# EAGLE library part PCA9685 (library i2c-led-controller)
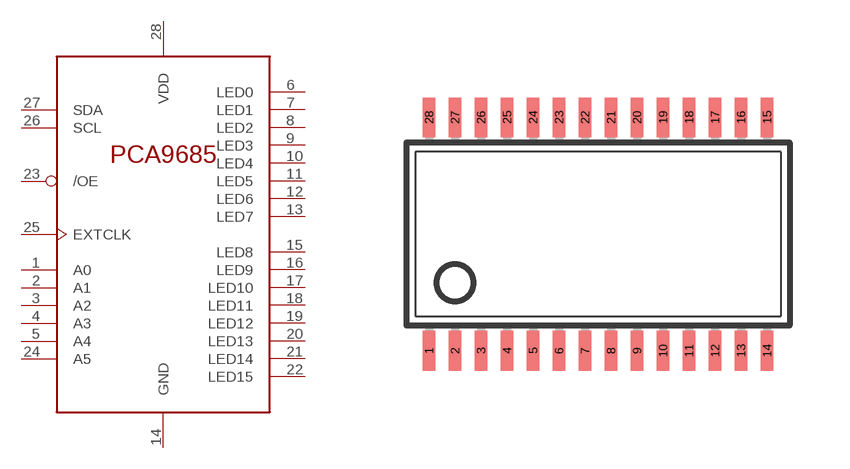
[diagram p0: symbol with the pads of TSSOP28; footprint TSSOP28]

Designator prefix -

## PCA9685PW  [TSSOP28]
1  A0
2  A1
3  A2
4  A3
5  A4
6  LED0
7  LED1
8  LED2
9  LED3
10  LED4
11  LED5
12  LED6
13  LED7
14  GND  pwr
15  LED8
16  LED9
17  LED10
18  LED11
19  LED12
20  LED13
21  LED14
22  LED15
23  /OE
24  A5
25  EXTCLK  in
26  SCL
27  SDA
28  VDD  pwr

## Footprint TSSOP28 (pad centres in mm)
smd 0.305 x 0.991: 1 -4.225,-2.918; 2 -3.575,-2.918; 3 -2.925,-2.918; 4 -2.275,-2.918; 5 -1.625,-2.918; 6 -0.975,-2.918; 7 -0.325,-2.918; 8 0.325,-2.918; 9 0.975,-2.918; 10 1.625,-2.918; 11 2.275,-2.918; 12 2.925,-2.918; 13 3.575,-2.918; 14 4.225,-2.918; 15 4.225,2.918; 16 3.575,2.918; 17 2.925,2.918; 18 2.275,2.918; 19 1.625,2.918; 20 0.975,2.918; 21 0.325,2.918; 22 -0.325,2.918; 23 -0.975,2.918; 24 -1.625,2.918; 25 -2.275,2.918; 26 -2.925,2.918; 27 -3.575,2.918; 28 -4.225,2.918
